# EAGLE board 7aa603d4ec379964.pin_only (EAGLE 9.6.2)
REV: B

Size 33.02 x 21.59 mm. Coordinates in mm from the lower left corner, seen from the top.
Outline: 33.02,2.54 33.02,19.05 arc90 30.48,21.59 2.54,21.59 arc90 0,19.05 0,2.54 arc90 2.54,0 30.48,0 arc90 33.02,2.54
Copper layers (1*16): Top 0.035mm / dielectric 1.5mm / Bottom 0.035mm
Design rules "adafruit *": minimum track width 8mil, minimum drill 15.5mil, track to track 8mil, track to pad 8mil, pad to pad 8mil, via to via 8mil, smd to smd 8mil, copper to edge 10mil, drill to drill 8mil, minimum pad ring 10mil, minimum via ring 8mil, stop-mask expansion 2mil, vias tented up to drill 20mil, thermal gap 10mil

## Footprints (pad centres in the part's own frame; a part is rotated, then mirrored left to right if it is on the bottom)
0603-NO = smd 1.075 x 1: 1 -0.85,0; 2 0.85,0
0805-NO = smd 1.24 x 1.5: 1 -0.95,0; 2 0.95,0
JST_SH4 = smd 0.6 x 1.55: 1 -1.5,2.514; 2 -0.5,2.514; 3 0.5,2.514; 4 1.5,2.514 | smd 1.2 x 1.8: MT1 -2.8,-1.386; MT2 2.8,-1.386
CHIPLED_0603_NOOUTLINE = smd 0.8 x 0.8: A 0,-0.75; C 0,0.75
SOD-323F = smd 1 x 0.8: A -1,0; C 1,0
FIDUCIAL_1MM = smd 1 x 1: 1 0,0
SOT23 = smd 1 x 1.4: 1 -0.95,-1.1; 2 0.95,-1.1; 3 0,1.1
1X06_ROUND_70 = drill 1 pad 1.778: 1 -6.35,0; 2 -3.81,0; 3 -1.27,0; 4 1.27,0; 5 3.81,0; 6 6.35,0
UG-2832HSWEG02_WRAPUNDER = smd 3.2 x 0.35 bottom: 1 -2.03,-5.3; 2 -2.03,-4.68; 3 -2.03,-4.06; 4 -2.03,-3.44; 5 -2.03,-2.82; 6 -2.03,-2.2; 7 -2.03,-1.58; 8 -2.03,-0.96; 9 -2.03,-0.34; 10 -2.03,0.28; 11 -2.03,0.9; 12 -2.03,1.52; 13 -2.03,2.14; 14 -2.03,2.76
SOT363 = smd 0.5 x 0.5: 1 -0.75,-0.9; 3 0.75,-0.9; 4 0.75,0.9; 6 -0.75,0.9 | smd 0.4 x 0.5: 2 0,-0.9; 5 0,0.9
RESPACK_4X0603 = smd 0.45 x 0.9: 1 -1.3,-0.85; 2 -0.4,-0.85; 3 0.4,-0.85; 4 1.3,-0.85; 5 1.3,0.85; 6 0.4,0.85; 7 -0.4,0.85; 8 -1.3,0.85
SOT23-5 = smd 0.55 x 1.2: 1 -0.95,-1.3; 2 0,-1.3; 3 0.95,-1.3; 4 0.95,1.3; 5 -0.95,1.3
MOUNTINGHOLE_2.5_PLATED = drill 2.5 pad 3.2: P$1 0,0

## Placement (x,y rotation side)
C1  0.1uF  [0603-NO]  19.94,6.98 270 top
C2  10uF  [0805-NO]  12.95,15.62 0 top
C3  10uF  [0805-NO]  14.86,9.02 0 top
C4  1uF  [0805-NO]  9.27,5.33 0 top
C5  1uF  [0805-NO]  9.27,7.24 180 top
C6  1uF  [0805-NO]  9.27,9.53 180 top
C7  1uF  [0805-NO]  9.27,11.43 180 top
C8  10uF  [0805-NO]  9.27,16.76 180 top
C9  10uF  [0805-NO]  9.27,14.86 180 top
CONN4  STEMMA_I2C_QT  [JST_SH4]  30.35,11.05 90 top
D1  GREEN  [CHIPLED_0603_NOOUTLINE]  31.37,6.48 90 top
D2  1N4148  [SOD-323F]  17.4,15.62 0 top
FID3  FIDUCIAL_1MM  [FIDUCIAL_1MM]  31.88,15.94 180 top
FID4  FIDUCIAL_1MM  [FIDUCIAL_1MM]  5.84,2.25 180 top
IC5  APX803  [SOT23]  17.4,11.3 180 top
JP1  [1X06_ROUND_70]  16.51,2.67 180 bottom
LCD1  [UG-2832HSWEG02_WRAPUNDER]  2.29,10.93 0 bottom
Q2  BSS138  [SOT363]  22.35,7.87 90 top
R1  10K  [0603-NO]  28.45,6.48 180 top
R2  390K  [0603-NO]  9.27,13.21 180 top
R3  10K  [RESPACK_4X0603]  22.35,12.07 270 top
R5  10K  [0603-NO]  17.4,14.1 0 top
U2  AP2112K-3.3  [SOT23-5]  12.95,12.19 180 top
U$1  MOUNTINGHOLE2.5  [MOUNTINGHOLE_2.5_PLATED]  30.48,2.54 180 top
U$17  MOUNTINGHOLE2.5  [MOUNTINGHOLE_2.5_PLATED]  2.54,2.54 180 top
U$19  MOUNTINGHOLE2.5  [MOUNTINGHOLE_2.5_PLATED]  30.48,19.05 180 top
U$21  MOUNTINGHOLE2.5  [MOUNTINGHOLE_2.5_PLATED]  2.54,19.05 180 top
U$22  [ADAFRUIT_3.5MM]  15.37,5.21 0 top
U$25  [PCBFEAT-REV-040]  5.84,17.65 180 top
U$31  [STEMMAQT]  24.26,14.73 270 top

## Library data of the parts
C1-C9 CONN4 D1 JP1 LCD1 Q2 R1-R3 R5 U2 U$22 U$25 = microbuilder
D2 IC5 = adafruit
FID3 FID4 U$1 U$17 U$19 U$21 = microbuilder; BOM: EXCLUDE
U$31 = silks

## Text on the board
tPlace: 0.91" OLED Display | 128x32 Monochrome / VLogic/Vin: 3-5VDC | I2C Addr 0x3C | on
bPlace: 0.91" OLED Display | 128x32 Monochrome | 3Vo | Reset | SDA | VIN | GND | SCL

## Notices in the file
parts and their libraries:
microbuilder: This work is placed in the public domain, and may be freely used for commercial and non-commercial work with the following conditions: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
